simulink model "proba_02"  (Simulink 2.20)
settings: Solver=FixedStepDiscrete  StartTime=0.0  StopTime=20.0  FixedStep=1  RelTol=1e-3  AbsTol=1e-6
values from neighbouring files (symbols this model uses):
  q0 = P+q2    [DPIDrc_S.m]    (also in PID01.m; ab2pq.m = 1.0/sum(B))
  q1 = -P+P*(h/I)-2*q2    [DPIDrc_S.m]    (also in PID01.m)
  q2 = P*(D/h)    [DPIDrc_S.m]    (also in PID01.m)

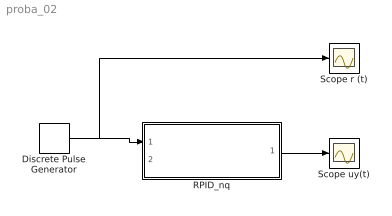
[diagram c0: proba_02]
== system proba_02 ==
  Discrete Pulse Generator : DiscretePulseGenerator  Amplitude=1  Period=20  PulseWidth=20  PhaseDelay=1  SampleTime=1
  RPID_nq : Subsystem  mask( PID ){P=1, I=25, D=1, h=1}
      mask prompts: I "I [s]:"; D "D [s]:"; h "h [s]:"
      mask help: PID : P, I, D - ; h - ;
      mask init:
      | %  Documentation
      |             P=@1;I=@2;D=@3;h=@4;
      | [q0,q1,q2]=pid01(P,I,D,h);
  Scope r (t) : Scope
  Scope uy(t) : Scope
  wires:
  Discrete Pulse Generator/1 -> Scope r (t)/1, RPID_nq/1(In1)
  RPID_nq/1(Out1) -> Scope uy(t)/1

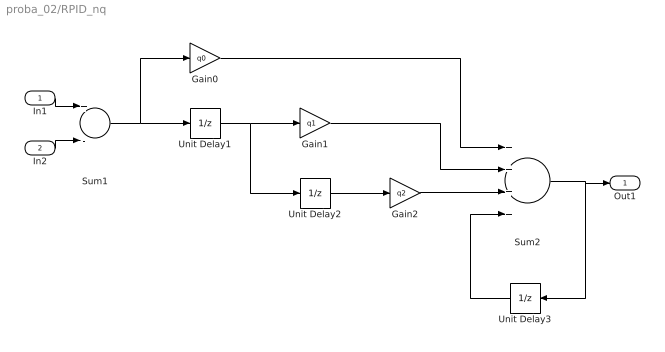
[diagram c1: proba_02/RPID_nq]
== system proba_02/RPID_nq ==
  In1 : Inport  Port=1  PortWidth=-1  SampleTime=-1
  In2 : Inport  Port=2  PortWidth=-1  SampleTime=-1
  Gain0 : Gain  Description=GAIN 0  Gain=q0
  Gain1 : Gain  Description=Gain 1  Gain=q1
  Gain2 : Gain  Gain=q2
  Sum1 : Sum  Inputs=+-
  Sum2 : Sum  Inputs=++++
  Unit Delay1 : UnitDelay  Description=Gain 0  X0=0  SampleTime=1
  Unit Delay2 : UnitDelay  Description=Gain 1  X0=0  SampleTime=1
  Unit Delay3 : UnitDelay  Orientation=left  X0=0  SampleTime=1
  Out1 : Outport  Port=1  InitialOutput=0
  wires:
  In2/1 -> Sum1/2
  In1/1 -> Sum1/1
  Unit Delay3/1 -> Sum2/4
  Sum2/1 -> Out1/1, Unit Delay3/1
  Gain2/1 -> Sum2/3
  Gain1/1 -> Sum2/2
  Unit Delay2/1 -> Gain2/1
  Unit Delay1/1 -> Unit Delay2/1, Gain1/1
  Gain0/1 -> Sum2/1
  Sum1/1 -> Gain0/1, Unit Delay1/1
